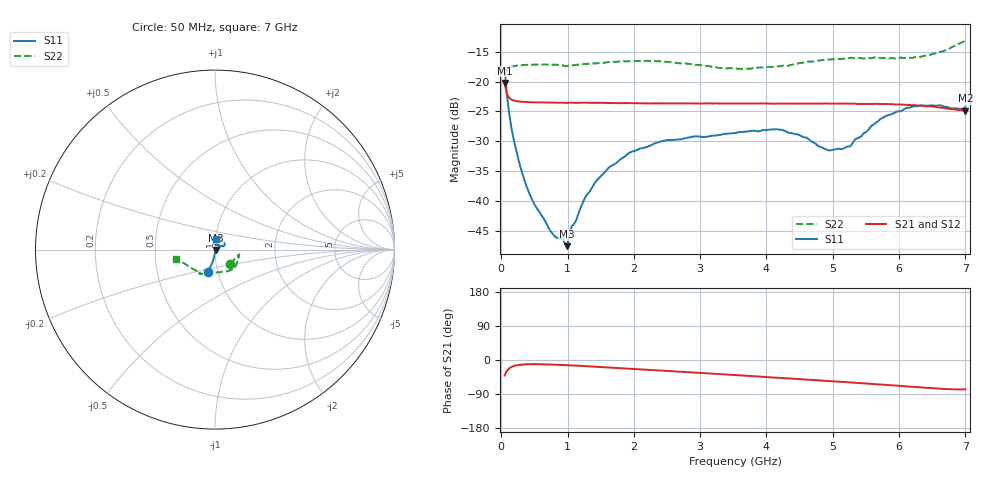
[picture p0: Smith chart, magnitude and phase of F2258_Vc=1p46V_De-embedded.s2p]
! Integrated Device Technology
! Corporate Headquarters
! 6024 Silver Creek Valley Road
! San Jose, CA 95138  USA
! Phone:  1-408-284-8200
! Toll Free:  1-800-223-1366
! Webpage:  http://www.idt.com/
! Timing and RF Division
! 515 Groton Road, Suite 102
! Westford, MA 01886-6024
! Device:  F2258
! Description: Voltage Variable RF Attenuator
! Frequency:  50.0 -  6000.00 MHz
! Package:  3x3 mm Thin QFN Plastic Package: 16 pin
! Ports:  2 RF, 2 DC
!  Pin  1  = NC
!  Pin  2  = NC
!  Pin  3  = RF2  = Port 2
!  Pin  4  = GND
!  Pin  5  = Vdd
!  Pin  6  = NC
!  Pin  7  = VCTRL
!  Pin  8  = NC
!  Pin  9  = GND
!  Pin 10  = RF1  = Port 1
!  Pin 11  = NC
!  Pin 12  = NC
!  Pin 13  = NC
!  Pin 14  = NC
!  Pin 15  = NC
!  Pin 16  = NC
! Vcntrl:  1.460 Volts
! Vdd:  +3.300 Volts
! Current:  1.161 mA
! Data:  The device was measured on a the F2258 evaluation board which has
!  individual transmission lines to the RF pins.  Data was collected
!  using a calibrated network analyzer.  The evaluation board was
!  de-embedded using a TRL calibration technique.
!  The reference plane is the edge of the package pin.
! Misc:  SN 10
!  Action Tracker AT0285
! Date Measured:  2014-12-10
! Date:  2016-01-13  MJV
! Note:
!  Integrated Device Technology supplies this data as a sample of measured
!  data at the package pin for this product.  Your particular data for this
!  product may vary.
!  Data was taken at 25 degrees C.
!  Integrated Device Technology reserves the right to change this data at anytime.
!Freq_(GHz)  S11M_(dB)  S11P_(deg)  S21M_(dB)  S21P_(deg)  S12M_(dB)  S12P_(deg)  S22M_(dB)  S22P_(deg)
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# GHz S dB R 50
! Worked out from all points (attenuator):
!   201 points, 50 MHz to 7 GHz, reference 50 ohm
!   highest |S21| = -20.23 dB at 50 MHz (marker M1); lowest = -24.9 dB at 7 GHz (marker M2)
!   lowest |S11| = -47.5 dB at 988.2 MHz (marker M3), VSWR 1.01, Z = 50.3 - j0.245 ohm
!   |S11| at or under -10 dB: start of sweep to end of sweep
!   |S22| runs from -18.9 to -13.1 dB; largest |S21 - S12| = 0.00027
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0.05  -17.72 -107.4  -20.23 -41.1  -20.23 -41.1  -18.89 -43.6
0.08475  -22.20 -101.9  -22.11 -28.8  -22.11 -28.8  -18.06 -22.5
0.15425  -27.87 -97.7  -23.04 -18.3  -23.03 -18.3  -17.53 -13.8
0.36275  -36.96 -88.4  -23.42 -11.5  -23.44 -11.5  -17.23 -11.7
0.50175  -40.57 -75.7  -23.50 -11.1  -23.50 -11.1  -17.17 -13.3
0.745  -45.06 -49.0  -23.52 -12.0  -23.53 -12.0  -17.22 -17.7
0.91875  -46.13 -7.8  -23.56 -13.2  -23.57 -13.2  -17.23 -21.6
0.98825  -47.55 -35.5  -23.56 -13.7  -23.56 -13.6  -17.42 -22.8
1.05775  -44.33 -15.7  -23.54 -14.2  -23.56 -14.2  -17.30 -23.9
1.2315  -40.23 3.1  -23.56 -15.7  -23.56 -15.7  -17.10 -27.2
1.44  -36.53 9.1  -23.57 -17.9  -23.55 -17.9  -16.96 -31.1
1.6485  -34.16 14.2  -23.58 -20.0  -23.60 -20.0  -16.74 -34.7
1.9265  -31.94 23.3  -23.62 -22.8  -23.62 -22.8  -16.61 -39.6
2.37825  -30.12 35.0  -23.65 -27.4  -23.65 -27.4  -16.62 -47.8
3.525  -28.62 85.3  -23.67 -39.7  -23.68 -39.7  -17.85 -81.0
4.1505  -27.99 102.7  -23.70 -46.6  -23.72 -46.6  -17.43 -103.3
4.7065  -30.17 92.6  -23.70 -52.8  -23.68 -52.8  -16.66 -115.2
4.94975  -31.54 74.0  -23.70 -55.6  -23.72 -55.5  -16.33 -117.7
5.2625  -30.86 44.4  -23.72 -59.2  -23.73 -59.1  -16.05 -120.3
5.85325  -25.60 23.5  -23.79 -66.4  -23.80 -66.4  -16.14 -125.9
6.33975  -23.95 30.5  -24.07 -72.7  -24.05 -72.8  -15.83 -138.1
7  -24.27 83.6  -24.86 -77.4  -24.85 -77.4  -13.13 -166.8
